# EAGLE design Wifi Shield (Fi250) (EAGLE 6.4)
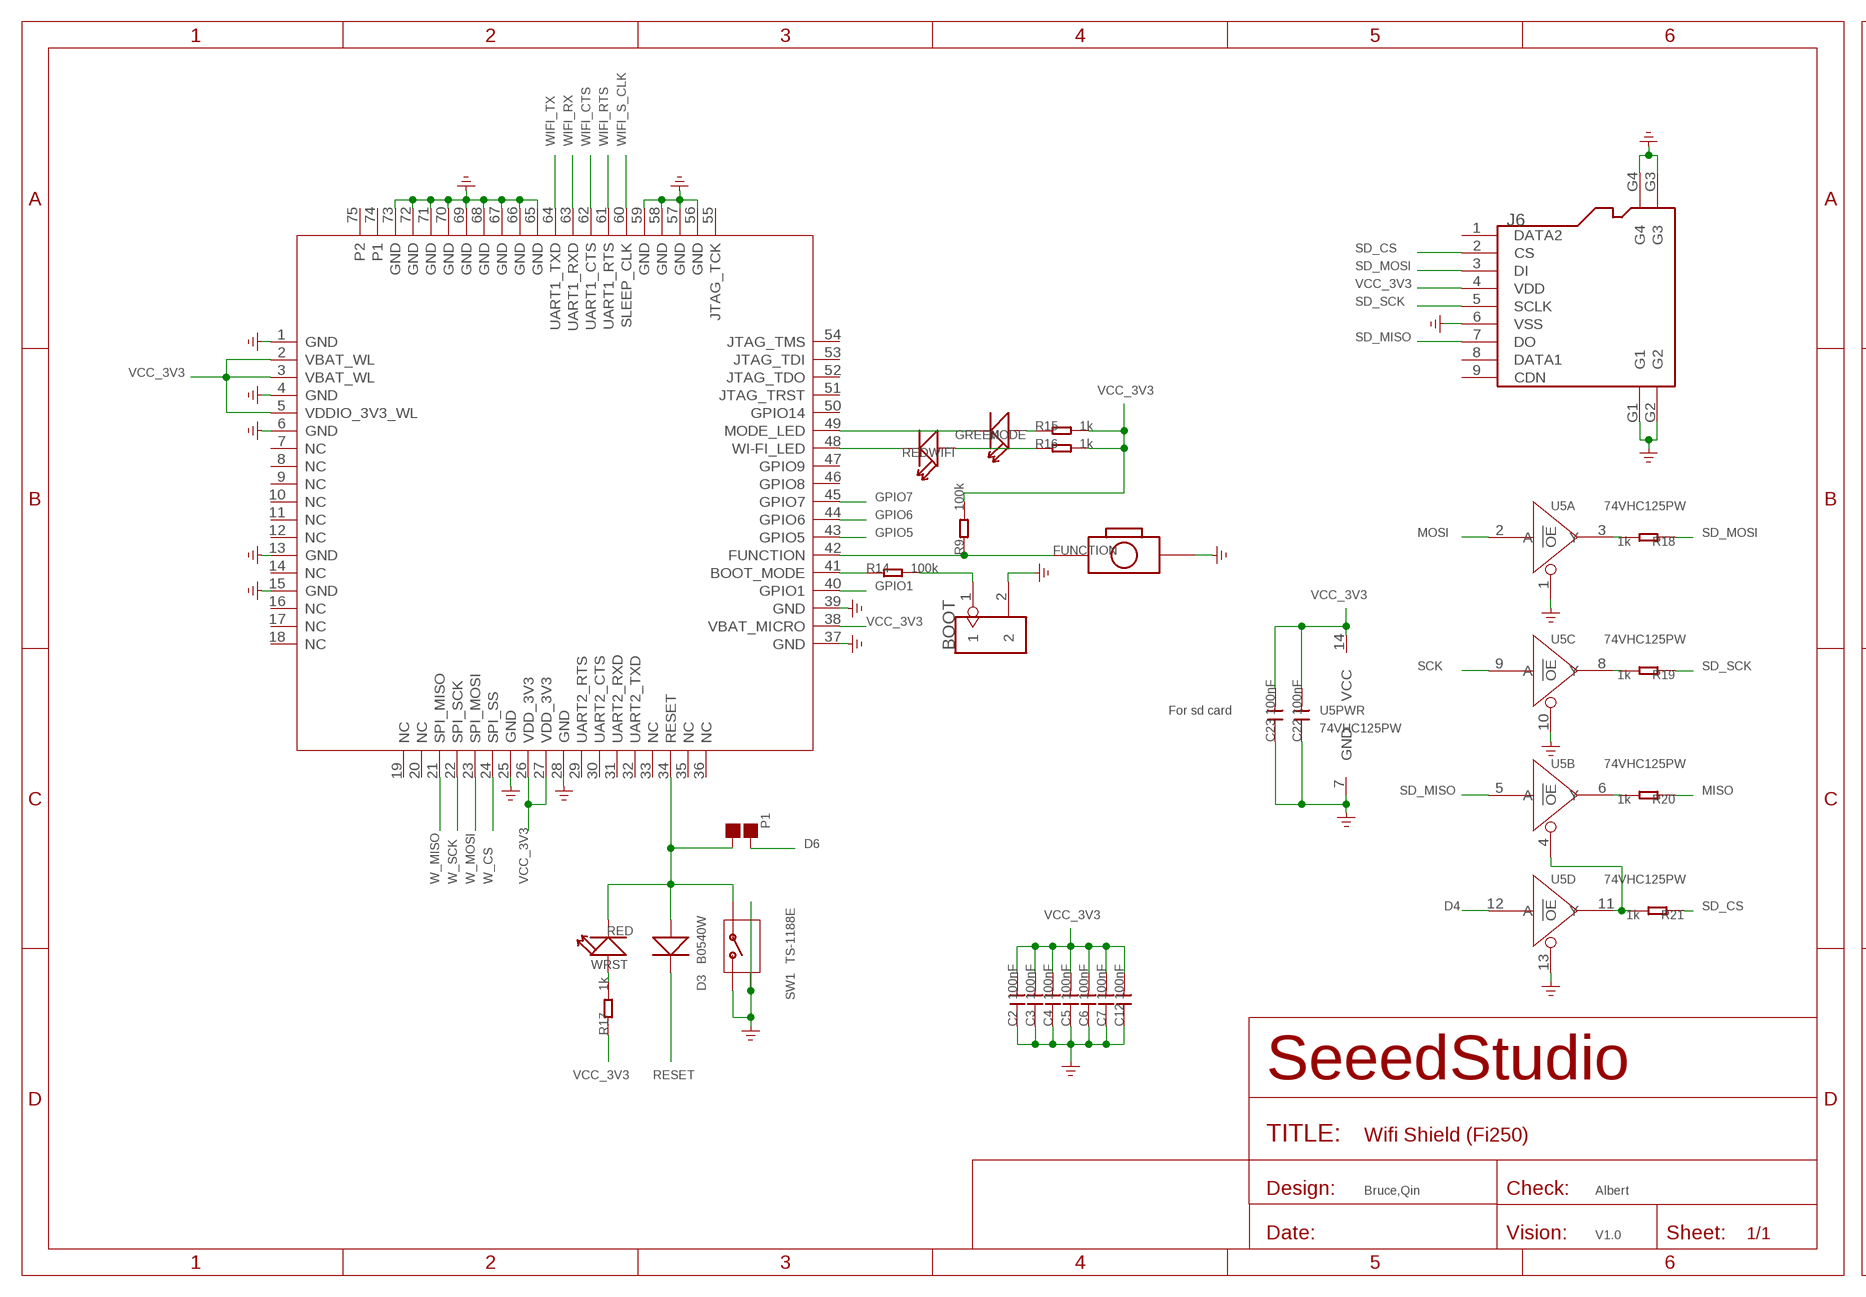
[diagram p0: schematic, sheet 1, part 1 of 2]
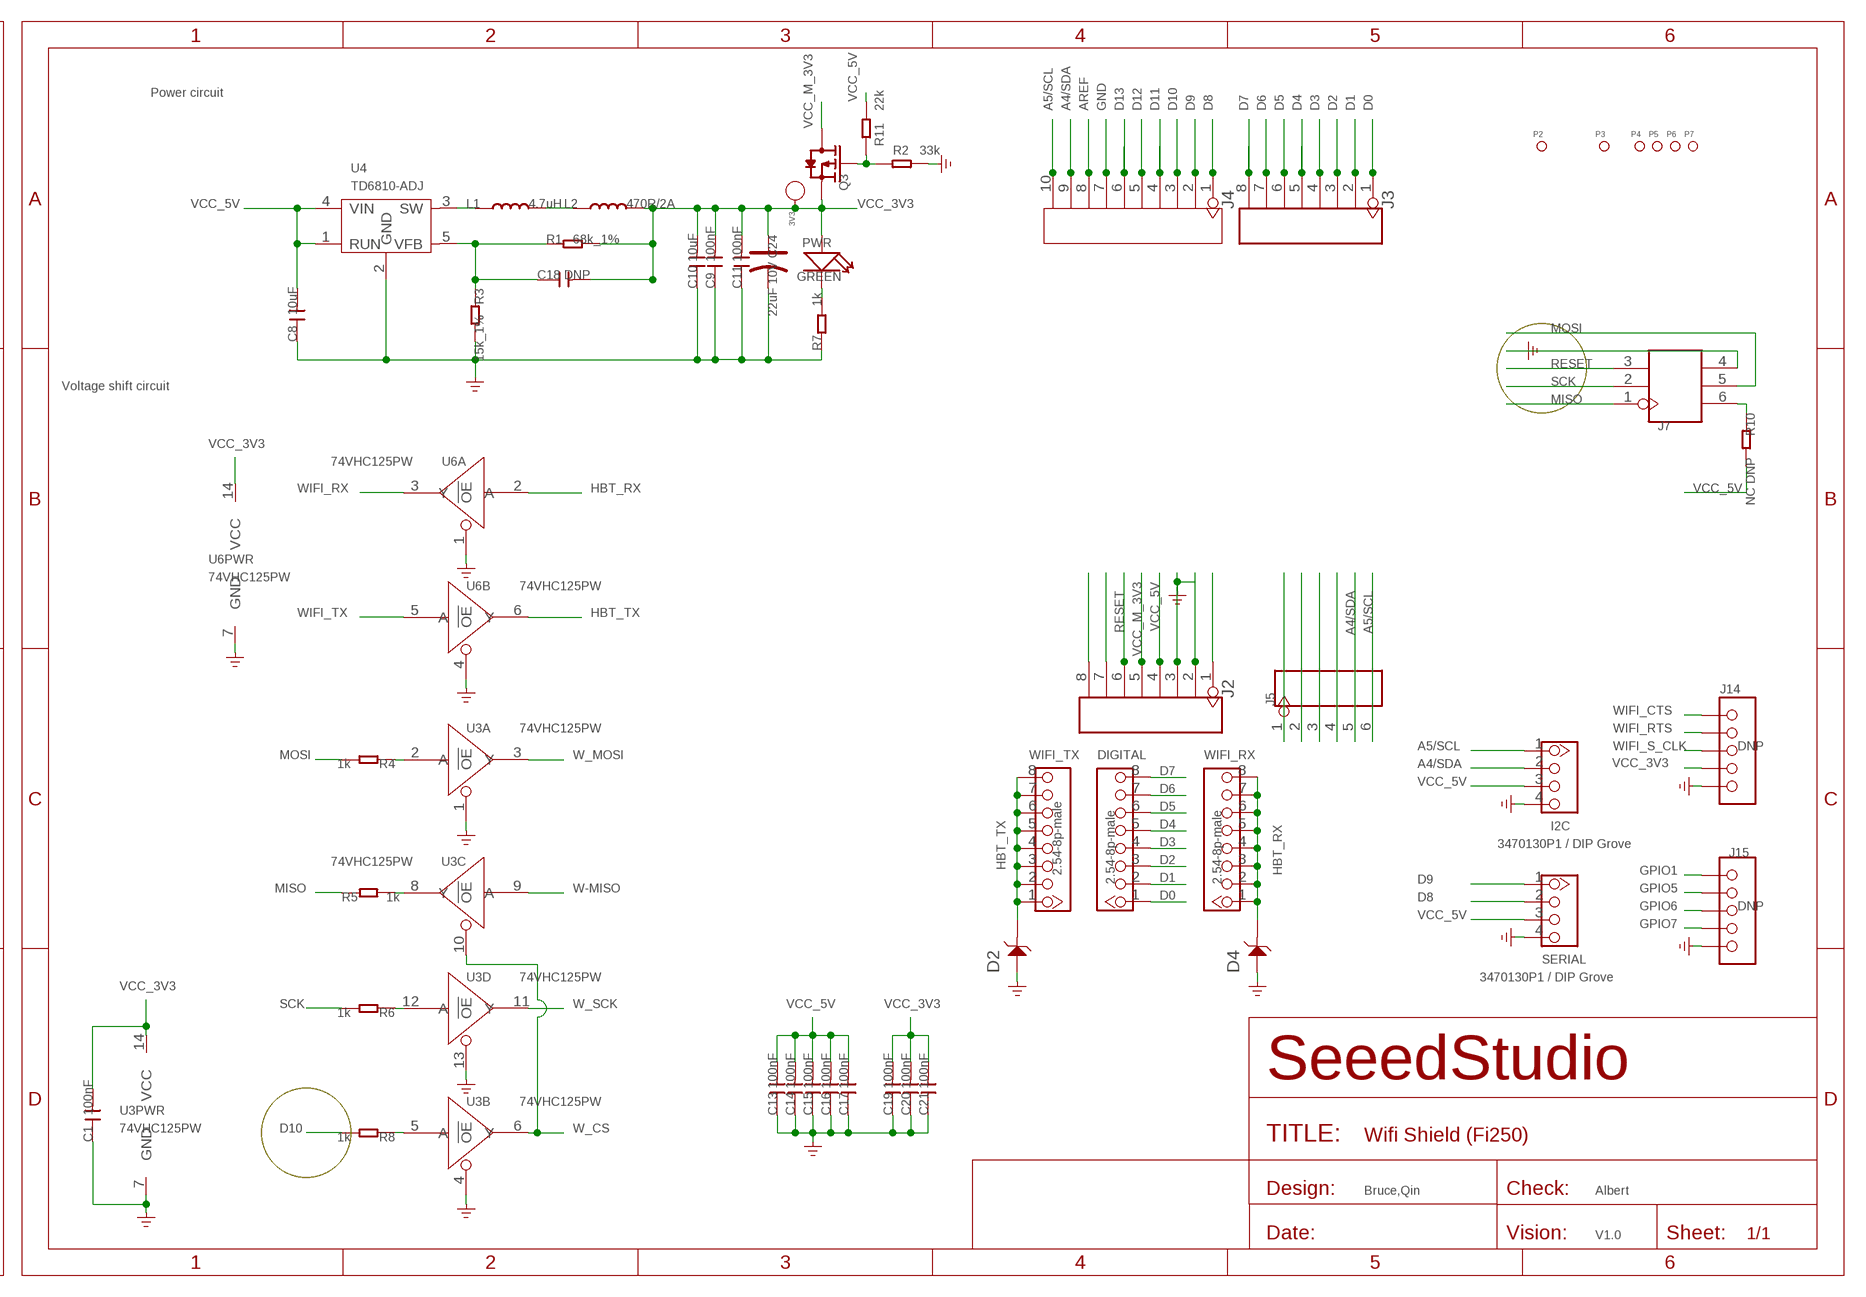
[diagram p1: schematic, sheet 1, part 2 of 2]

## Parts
3V3  PAD-TEST-POINT'4545'  [TP_4545]
BOOT  HEADER-2P-65/35MIL  [2P-2.54-65/35MIL]
C1  100nF  C-0603  [C0603]
C2  100nF  C-0603  [C0603]
C3  100nF  C-0603  [C0603]
C4  100nF  C-0603  [C0603]
C5  100nF  C-0603  [C0603]
C6  100nF  C-0603  [C0603]
C7  100nF  C-0603  [C0603]
C8  10uF  C-0805  [C0805]
C9  100nF  C-0603  [C0603]
C10  10uF  C-0805  [C0805]
C11  100nF  C-0603  [C0603]
C12  100nF  C-0603  [C0603]
C13  100nF  C-0603  [C0603]
C14  100nF  C-0603  [C0603]
C15  100nF  C-0603  [C0603]
C16  100nF  C-0603  [C0603]
C17  100nF  C-0603  [C0603]
C18  DNP  C-0603  [C0603]
C19  100nF  C-0603  [C0603]
C20  100nF  C-0603  [C0603]
C21  100nF  C-0603  [C0603]
C22  100nF  C-0603  [C0603]
C23  100nF  C-0603  [C0603]
C24  22uF 10V  CAP-AVX-A  [AVX-A]
D2  D-ESD-2P'CESD5V0D1'  [SOD123-2.7X1.6]
D3  B0540W  D'1206'  [SOD123]
D4  D-ESD-2P'CESD5V0D1'  [SOD123-2.7X1.6]
DIGITAL  2.54-8p-male  HEADER-8P-2.54  [8P-2.54]
FUNCTION  BUTTON-2P-SMD  [2P-SMD-6.1X3.81]
I2C  3470130P1 / DIP Grove  TWIG-4P-2.0-2.0  [4P-2.0]
J2  HEADER-8P-65/35MIL  [8P-2.54-65/35MIL]
J3  HEADER-8P-65/35MIL  [8P-2.54-65/35MIL]
J4  HEADER-10P-2.54  [10P-2.54]
J5  HEADER-6P-65/35MIL  [6P-2.54-65/35MIL]
J6  HOLDER-MICROSD-9P  [9P-SMD-W/-RING]
J7  HEADER-2X3P-65/35MIL  [2X3P-2.54-65/35MIL]
J14  DNP  HEADER-5P-2.54  [5P-2.54]
J15  DNP  HEADER-5P-2.54  [5P-2.54]
L1  4.7uH  LSPD3D16-4R7M  [L0420]
L2  470R/2A  L'0805'  [L0805]
MODE  GREEN  LED'0603'  [LED-0603]
P1  DNP  PAD-JUMPER-2P  [2P-SMD-1.78X1.27]
P2  PAD-MARK  [ROUND-MARK-1.0]
P3  PAD-MARK  [ROUND-MARK-1.0]
P4  PAD-MARK  [ROUND-MARK-1.0]
P5  PAD-MARK  [ROUND-MARK-1.0]
P6  PAD-MARK  [ROUND-MARK-1.0]
P7  PAD-MARK  [ROUND-MARK-1.0]
PWR  GREEN  LED'0603'  [LED-0603]
Q3  MOSFET-P'SI2323CDS/SI2305DS<BR>'  [SOT23]
R1  68k_1%  R-0603  [R0603]
R2  33k  R-0603  [R0603]
R3  15k_1%  R-0603  [R0603]
R4  1k  R-0603  [R0603]
R5  1k  R-0603  [R0603]
R6  1k  R-0603  [R0603]
R7  1k  R-0603  [R0603]
R8  1k  R-0603  [R0603]
R9  100k  R-0603  [R0603]
R10  NC DNP  R-0603  [R0603]
R11  22k  R-0603  [R0603]
R14  100k  R-0603  [R0603]
R15  1k  R-0603  [R0603]
R16  1k  R-0603  [R0603]
R17  1k  R-0603  [R0603]
R18  1k  R-0603  [R0603]
R19  1k  R-0603  [R0603]
R20  1k  R-0603  [R0603]
R21  1k  R-0603  [R0603]
SERIAL  3470130P1 / DIP Grove  TWIG-4P-2.0-2.0  [4P-2.0]
SW1  TS-1188E  BUTTON-4P-REINFORCE'TS-1188E'  [4P-SMD-7X3.5X3.5H]
U1  WIZFI250  [73P-28X20MM]
U3  74VHC125PW  74VHCT125PW  [TSSOP14]
U4  TD6810-ADJ  TD6810'TSOT23-5'  [SOT23-5]
U5  74VHC125PW  [TSSOP14]
U6  74VHC125PW  [TSSOP14]
WIFI  RED  LED'0603'  [LED-0603]
WIFI_RX  2.54-8p-male  HEADER-8P-2.54  [8P-2.54]
WIFI_TX  2.54-8p-male  HEADER-8P-2.54  [8P-2.54]
WRST  RED  LED'0603'  [LED-0603]

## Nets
A4/SDA: I2C.2 J4.9 J5.5
A5/SCL: I2C.1 J4.10 J5.6
AREF: J4.8
D0: DIGITAL.1 J3.1
D1: DIGITAL.2 J3.2
D2: DIGITAL.3 J3.3
D3: DIGITAL.4 J3.4
D4: DIGITAL.5 J3.5 U5.12(D:A)
D5: DIGITAL.6 J3.6
D6: DIGITAL.7 J3.7 P1.2
D7: DIGITAL.8 J3.8
D8: J4.1 SERIAL.2
D9: J4.2 SERIAL.1
D10: J4.3 R8.2
D11: J4.4
D12: J4.5
D13: J4.6
GND: BOOT.2 C1.1 C2.1 C3.1 C4.1 C5.1 C6.1 C7.1 C8.1 C9.1 C10.1 C11.1 C12.1 C13.1 C14.1 C15.1 C16.1 C17.1 C19.1 C20.1 C21.1 C22.1 C23.1 C24.- D2.1 D4.1 FUNCTION.P$2 I2C.4 J2.2 J2.3 J4.7 J6.6(VSS) J6.G1 J6.G2 J6.G3 J6.G4 J7.4 J14.5 J15.5 R2.1 R3.2 R7.1 SERIAL.4 SW1.2 SW1.S1 SW1.S2 U1.1(GND) U1.4(GND) U1.6(GND) U1.13(GND) U1.15(GND) U1.25(GND) U1.28(GND) U1.37(GND) U1.39(GND) U1.56(GND) U1.57(GND) U1.58(GND) U1.59(GND) U1.65(GND) U1.66(GND) U1.67(GND) U1.68(GND) U1.69(GND) U1.70(GND) U1.71(GND) U1.72(GND) U1.73(GND) U3.1(A:!OE) U3.4(B:!OE) U3.7(PWR:GND) U3.13(D:!OE) U4.2(GND) U5.1(A:!OE) U5.7(PWR:GND) U5.10(C:!OE) U5.13(D:!OE) U6.1(A:!OE) U6.4(B:!OE) U6.7(PWR:GND)
GPIO1: J15.1 U1.40(GPIO1)
GPIO5: J15.2 U1.43(GPIO5)
GPIO6: J15.3 U1.44(GPIO6)
GPIO7: J15.4 U1.45(GPIO7)
HBT_RX: D4.2 U6.2(A:A) WIFI_RX.1 WIFI_RX.2 WIFI_RX.3 WIFI_RX.4 WIFI_RX.5 WIFI_RX.6 WIFI_RX.7 WIFI_RX.8
HBT_TX: D2.2 U6.6(B:Y) WIFI_TX.1 WIFI_TX.2 WIFI_TX.3 WIFI_TX.4 WIFI_TX.5 WIFI_TX.6 WIFI_TX.7 WIFI_TX.8
MISO: J7.1 R5.1 R20.1
MOSI: J7.5 R4.2 U5.2(A:A)
N$1: J2.1
N$2: J2.7
N$3: R4.1 U3.2(A:A)
N$4: R6.1 U3.12(D:A)
N$5: J7.6 R10.1
N$6: R5.2 U3.8(C:Y)
N$7: FUNCTION.1 R9.1 U1.42(FUNCTION)
N$8: L1.1 U4.3(SW)
N$9: R17.2 WRST.+
N$10: L1.2 L2.1
N$11: J2.8
N$12: MODE.- U1.49(MODE_LED)
N$13: U1.48(WI-FI_LED) WIFI.-
N$14: BOOT.1 R14.2
N$15: R16.1 WIFI.+
N$16: J5.1
N$17: J5.2
N$18: MODE.+ R15.1
N$19: R14.1 U1.41(BOOT_MODE)
N$20: D3.+ P1.1 SW1.1 U1.34(RESET) WRST.-
N$21: J5.3
N$22: J5.4
N$23: Q3.1(G) R2.2 R11.2
N$24: R18.2 U5.3(A:Y)
N$26: PWR.- R7.2
N$27: R8.1 U3.5(B:A)
N$28: R19.2 U5.8(C:Y)
N$29: R20.2 U5.6(B:Y)
N$30: R21.2 U5.4(B:!OE) U5.11(D:Y)
N$39: C18.1 R1.1 R3.1 U4.5(VFB)
RESET: D3.- J2.6 J7.3
SCK: J7.2 R6.2 U5.9(C:A)
SD_CS: J6.2(CS) R21.1
SD_MISO: J6.7(DO) U5.5(B:A)
SD_MOSI: J6.3(DI) R18.1
SD_SCK: J6.5(SCLK) R19.1
VCC_3V3: 3V3.T C1.2 C2.2 C3.2 C4.2 C5.2 C6.2 C7.2 C9.2 C10.2 C11.2 C12.2 C18.2 C19.2 C20.2 C21.2 C22.2 C23.2 C24.+ J6.4(VDD) J14.4 L2.2 PWR.+ Q3.2(S) R1.2 R9.2 R15.2 R16.2 R17.1 U1.2(VBAT_WL) U1.3(VBAT_WL) U1.5(VDDIO_3V3_WL) U1.26(VDD_3V3) U1.27(VDD_3V3) U1.38(VBAT_MICRO) U3.14(PWR:VCC) U5.14(PWR:VCC) U6.14(PWR:VCC)
VCC_5V: C8.2 C13.2 C14.2 C15.2 C16.2 C17.2 I2C.3 J2.4 R10.2 R11.1 SERIAL.3 U4.1(RUN) U4.4(VIN)
VCC_M_3V3: J2.5 Q3.3(D)
W-MISO: U3.9(C:A)
W_CS: U1.24(SPI_SS) U3.6(B:Y) U3.10(C:!OE)
W_MISO: U1.21(SPI_MISO)
W_MOSI: U1.23(SPI_MOSI) U3.3(A:Y)
W_SCK: U1.22(SPI_SCK) U3.11(D:Y)
WIFI_CTS: J14.1 U1.62(UART1_CTS)
WIFI_RTS: J14.2 U1.61(UART1_RTS)
WIFI_RX: U1.63(UART1_RXD) U6.3(A:Y)
WIFI_S_CLK: J14.3 U1.60(SLEEP_CLK)
WIFI_TX: U1.64(UART1_TXD) U6.5(B:A)
Unconnected: J6.1(DATA2) J6.8(DATA1) J6.9(CDN) U1.7(NC) U1.8(NC) U1.9(NC) U1.10(NC) U1.11(NC) U1.12(NC) U1.14(NC) U1.16(NC) U1.17(NC) U1.18(NC) U1.19(NC) U1.20(NC) U1.29(UART2_RTS) U1.30(UART2_CTS) U1.31(UART2_RXD) U1.32(UART2_TXD) U1.33(NC) U1.35(NC) U1.36(NC) U1.46(GPIO8) U1.47(GPIO9) U1.50(GPIO14) U1.51(JTAG_TRST) U1.52(JTAG_TDO) U1.53(JTAG_TDI) U1.54(JTAG_TMS) U1.55(JTAG_TCK) U1.74(P1) U1.75(P2) U6.8(C:Y) U6.9(C:A) U6.10(C:!OE) U6.11(D:Y) U6.12(D:A) U6.13(D:!OE)

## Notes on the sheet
- Power circuit
- Voltage shift circuit
- For sd card
- Bruce,Qin | Albert | Bruce,Qin | Albert
- V1.0 | V1.0

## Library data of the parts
3V3 = Discrete:PAD-TEST-POINT; PARTNO: DNP
BOOT = Connector :HEADER-2P
C1-C23 = Discrete:C*: Ceramic Capacitors
C24 = Discrete:CAP*: Electrolytic Capacitors,Tantalum Capacitors and Super Capacitors
D2 D4 = Discrete:D-ESD-2P: Diodes for Protectiong against ESD
D3 = Discrete:D*
DIGITAL WIFI_RX WIFI_TX = Connector:HEADER-8P
FUNCTION = Discrete:BUTTON-2P
I2C SERIAL = Connector:TWIG-4P-2.0
J2 J3 = Connector :HEADER-8P
J4 = Connector :HEADER-10P
J5 = Connector :HEADER-6P
J6 = Connector :HOLDER-MICROSD-9P
J7 = Connector :HEADER-2X3P
J14 J15 = Connector:HEADER-5P
L1 = template:L
L2 = Discrete:L*
MODE PWR WIFI WRST = Discrete:LED*
P1 = Discrete:PAD-JUMPER-2P; PARTNO: DNP
P2-P7 = Discrete:PAD-MARK; PARTNO: DNP
Q3 = Discrete:MOSFET-P
R1-R11 R14-R21 = Discrete:R*
SW1 = Discrete:BUTTON-4P-REINFORCE: TS-1188E http://www.best-dz.com/?thread-374-2.html
U1 = template:WIZFI250: The WizFi250 provides for the highest-level integration, featuring 802.11b/g and 802.11n. It includes a 2.4 GHz WLAN CMOS power amplifier (PA) that meets the output power requirements of most handheld systems.
U3 U5 U6 = IC:74V*125: Quad Buffer/Line Driver;3-state
U4 = template:TD6810: 1.5MHz 800mA Synchronous Step-Down Regulator Dropout http://www.techcodeok.com/download/TD6810.pdf

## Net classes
0 default: width 0.152 mm, drill 0.305 mm, clearance 0.152 mm

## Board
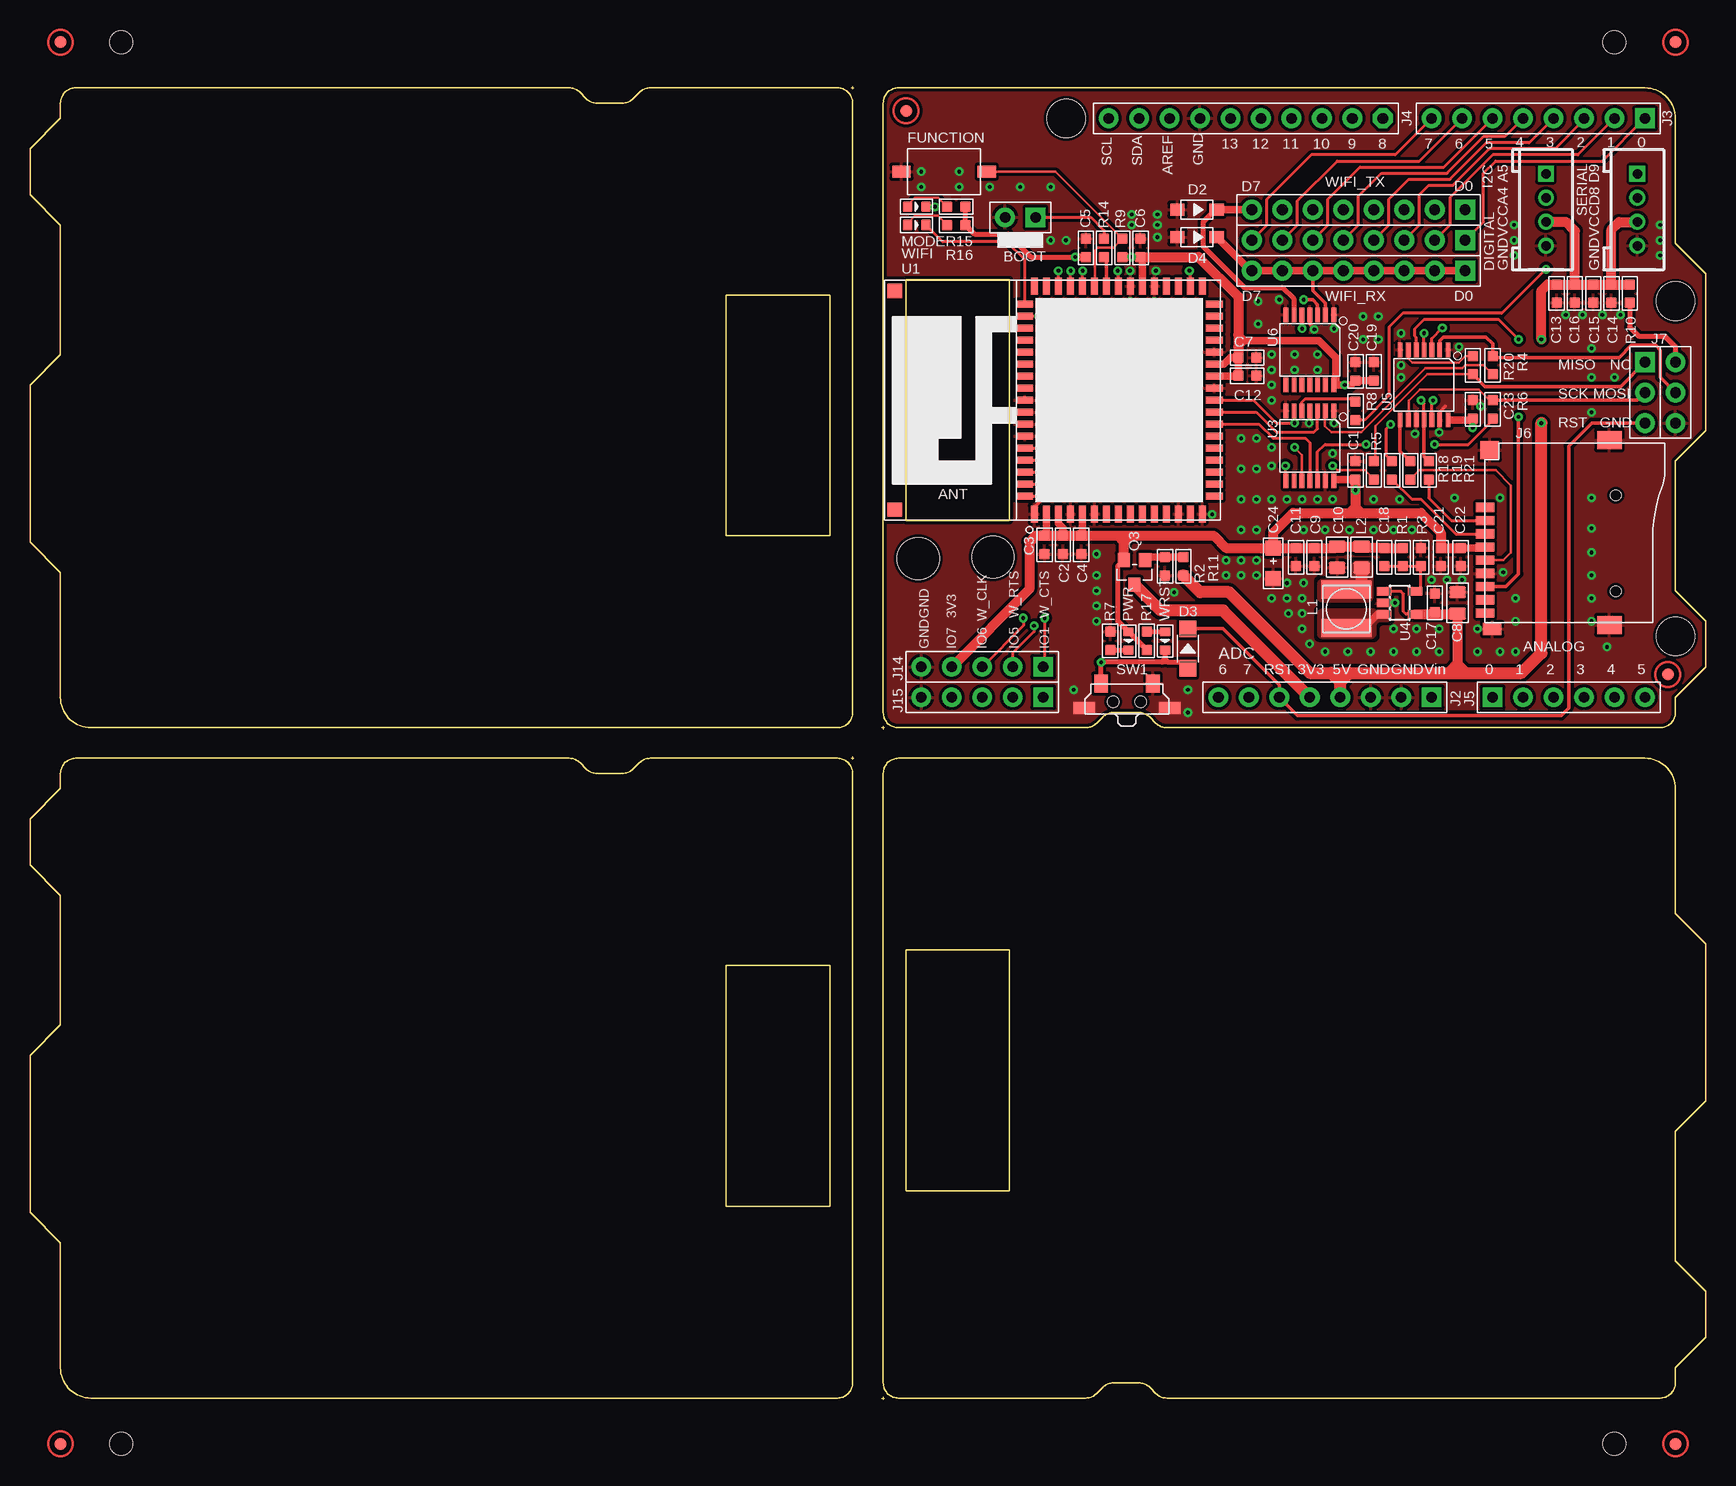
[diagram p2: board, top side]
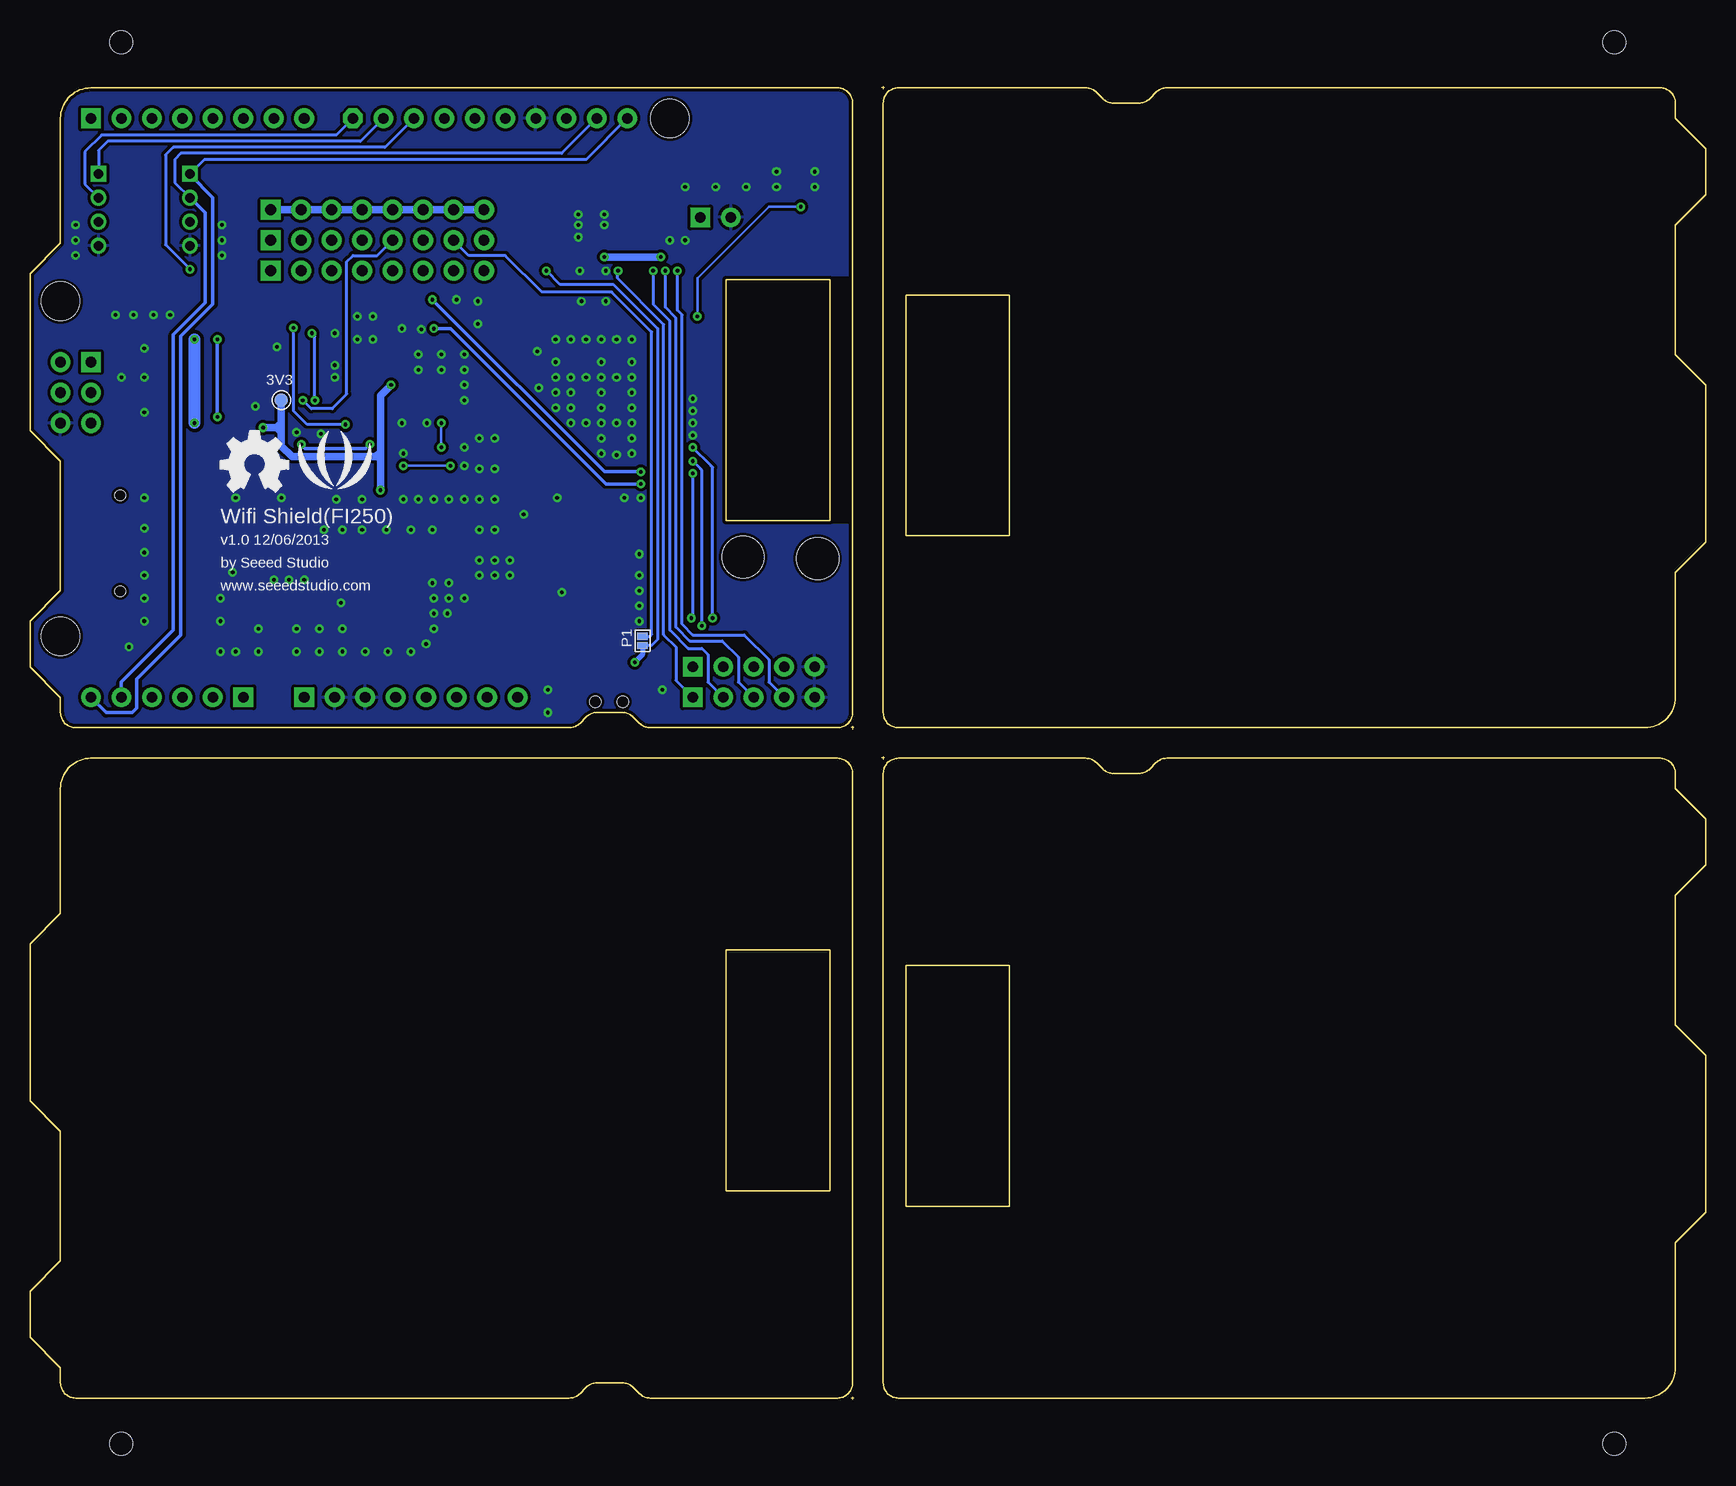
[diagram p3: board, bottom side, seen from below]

Size 139.7 x 109.47 mm. Coordinates in mm from the lower left corner, seen from the top.
Outline: 120 segments
Copper layers (1*16): Top 0.035mm / dielectric 1.5mm / Bottom 0.035mm
Design rules "default *": minimum track width 6mil, minimum drill 12mil, track to track 8mil, track to pad 8mil, pad to pad 8mil, via to via 8mil, smd to smd 0mil, copper to edge 10mil, drill to drill 8mil, minimum pad ring 10mil, minimum via ring 8mil, stop-mask expansion 4mil, vias tented up to drill 100mil, thermal gap 10mil
Holes 3.5 mm at 80.26,70.23 74.04,70.1
Holes 3.2 mm at 86.36,106.81 137.16,63.63 137.16,91.57
Holes 1.91 mm at 7.62,113.16 132.08,113.16 132.08,-3.68 7.62,-3.68
tRestrict: area 82.7,82.8 to 83.3,82.9; area 82.7,81.8 to 83.3,81.9; area 82.7,80.8 to 83.3,80.9

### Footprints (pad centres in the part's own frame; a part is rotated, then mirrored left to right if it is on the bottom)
TP_4545 = smd 1.143 x 1.143: T 0,0
2P-2.54-65/35MIL = drill 0.889 pad 1.651 square: 1 0,1.27 | drill 0.889 pad 1.651: 2 0,-1.27
C0603 = smd 0.889 x 0.889: 1 -0.762,0; 2 0.762,0
C0805 = smd 1.016 x 1.397: 1 -0.889,0; 2 0.889,0
AVX-A = smd 1.27 x 1.27: + -1.27,0; - 1.27,0
SOD123-2.7X1.6 = smd 1.2 x 1.02: 1 -1.635,0; 2 1.635,0
SOD123 = smd 1.397 x 1.397: + -1.651,0; - 1.651,0
8P-2.54 = drill 0.889 pad 1.651 square: 1 0,8.89 | drill 0.889 pad 1.651: 2 0,6.35; 3 0,3.81; 4 0,1.27; 5 0,-1.27; 6 0,-3.81; 7 0,-6.35; 8 0,-8.89
2P-SMD-6.1X3.81 = smd 1.524 x 1.016: 1 -3.556,0; P$2 3.556,0
4P-2.0 = drill 0.8 pad 1.27 square: 1 -3,0 | drill 0.8 pad 1.27: 2 -1,0; 3 1,0; 4 3,0
8P-2.54-65/35MIL = drill 0.889 pad 1.651 square: 1 0,8.89 | drill 0.889 pad 1.651: 2 0,6.35; 3 0,3.81; 4 0,1.27; 5 0,-1.27; 6 0,-3.81; 7 0,-6.35; 8 0,-8.89
10P-2.54 = drill 0.889 pad 1.651 octagon: 1 0,11.43 | drill 0.889 pad 1.651: 2 0,8.89; 3 0,6.35; 4 0,3.81; 5 0,1.27; 6 0,-1.27; 7 0,-3.81; 8 0,-6.35; 9 0,-8.89; 10 0,-11.43
6P-2.54-65/35MIL = drill 0.889 pad 1.651 square: 1 0,6.35 | drill 0.889 pad 1.651: 2 0,3.81; 3 0,1.27; 4 0,-1.27; 5 0,-3.81; 6 0,-6.35
9P-SMD-W/-RING = smd 1.524 x 0.762: 1 0,4.4; 2 0,3.3; 3 0,2.2; 4 0,1.1; 5 0,0; 6 0,-1.1; 7 0,-2.2; 8 0,-3.3; 9 0,-4.4 | smd 1.524 x 1.016: G1 0.6,-5.746 | smd 2.032 x 1.524: G2 10.373,-5.4; G3 10.373,10 | smd 1.524 x 1.524: G4 0.392,9.181 | hole 0.889: 10.9,-2.6; 10.9,5.4
2X3P-2.54-65/35MIL = drill 0.889 pad 1.651 square: 1 -1.27,2.54 | drill 0.889 pad 1.651: 2 -1.27,0; 3 -1.27,-2.54; 4 1.27,-2.54; 5 1.27,0; 6 1.27,2.54
5P-2.54 = drill 0.889 pad 1.651 square: 1 0,5.08 | drill 0.889 pad 1.651: 2 0,2.54; 3 0,0; 4 0,-2.54; 5 0,-5.08
L0420 = smd 1.5 x 4.2: 1 -1.6,0; 2 1.6,0
L0805 = smd 1.016 x 1.397: 1 -0.889,0; 2 0.889,0
LED-0603 = smd 0.762 x 0.889: + -0.762,0; - 0.762,0
2P-SMD-1.78X1.27 = smd 0.889 x 0.61: 1 0,0.381; 2 0,-0.381
ROUND-MARK-1.0 = smd 1.016 x 1.016: P$1 0,0
SOT23 = smd 1.016 x 1.143: 1 -0.889,-1.016; 2 0.889,-1.016; 3 0,1.016
R0603 = smd 0.889 x 0.889: 1 -0.762,0; 2 0.762,0
4P-SMD-7X3.5X3.5H = smd 1.143 x 1.524: 1 -2.159,1.524; 2 2.159,1.524 | smd 1.778 x 1.016: S1 -3.556,-0.508; S2 3.556,-0.508 | hole 0.95: -1.15,0; 1.15,0
73P-28X20MM = smd 0.6 x 1.4: 1 -1.5,-9.5; 2 -0.5,-9.5; 3 0.5,-9.5; 4 1.5,-9.5; 5 2.5,-9.5; 6 3.5,-9.5; 7 4.5,-9.5; 8 5.5,-9.5; 9 6.5,-9.5; 10 7.5,-9.5; 11 8.5,-9.5; 12 9.5,-9.5; 13 10.5,-9.5; 14 11.5,-9.5; 15 12.5,-9.5; 33 12.5,9.5; 34 11.5,9.5; 35 10.5,9.5; 36 9.5,9.5; 37 8.5,9.5; 38 7.5,9.5; 39 6.5,9.5; 40 5.5,9.5; 41 4.5,9.5; 42 3.5,9.5; 43 2.5,9.5; 44 1.5,9.5; 45 0.5,9.5; 46 -0.5,9.5; 47 -1.5,9.5 | smd 1.4 x 0.6: 16 13.5,-8; 17 13.5,-7; 18 13.5,-6; 19 13.5,-5; 20 13.5,-4; 21 13.5,-3; 22 13.5,-2; 23 13.5,-1; 24 13.5,0; 25 13.5,1; 26 13.5,2; 27 13.5,3; 28 13.5,4; 29 13.5,5; 30 13.5,6; 31 13.5,7; 32 13.5,8; 48 -2.3,8; 49 -2.3,7; 50 -2.3,6; 51 -2.3,5; 52 -2.3,4; 53 -2.3,3; 54 -2.3,2; 55 -2.3,1; 56 -2.3,0; 57 -2.3,-1; 58 -2.3,-2; 59 -2.3,-3; 60 -2.3,-4; 61 -2.3,-5; 62 -2.3,-6; 63 -2.3,-7; 64 -2.3,-8 | smd 1.2 x 1.2: 65 2.5,-3.5; 66 5.5,-3.5; 67 8.5,-3.5; 68 2.5,0; 69 5.5,0; 70 8.5,0; 71 2.5,3.5; 72 5.5,3.5; 73 8.5,3.5; 74 -13.12,9.12; 75 -13.12,-9.12
TSSOP14 = smd 0.4 x 1.2: 1 -2,-2.925; 2 -1.3,-2.925; 3 -0.65,-2.925; 4 0,-2.925; 5 0.65,-2.925; 6 1.3,-2.925; 7 2,-2.925; 8 2,2.925; 9 1.3,2.925; 10 0.65,2.925; 11 0,2.925; 12 -0.65,2.925; 13 -1.3,2.925; 14 -2,2.925
SOT23-5 = smd 0.69 x 1.2: 1 -0.95,-1.3; 2 0,-1.3; 3 0.95,-1.3; 4 0.95,1.3; 5 -0.95,1.3

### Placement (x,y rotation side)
3V3  118.75,83.31 0 bottom
BOOT  82.55,98.55 270 top
C1  110.49,77.47 270 top
C2  86.11,71.25 90 top
C3  84.58,71.25 90 top
C4  87.63,71.25 90 top
C5  88.01,96.01 270 top
C6  92.58,96.01 270 top
C7  101.47,86.87 180 top
C8  119,66.42 270 top
C9  107.06,70.23 90 top
C10  108.97,70.23 90 top
C11  105.54,70.23 90 top
C12  101.47,85.34 180 top
C13  127.25,92.2 90 top
C14  131.83,92.2 90 top
C15  130.3,92.2 90 top
C16  128.78,92.2 90 top
C17  117.09,66.42 270 top
C18  112.9,70.23 90 top
C19  112.01,85.72 270 top
C20  110.49,85.72 270 top
C21  117.6,70.23 90 top
C22  119.25,70.23 90 top
C23  120.27,82.55 270 top
C24  103.63,69.72 270 top
D2  97.28,99.19 0 top
D3  96.52,62.61 90 top
D4  97.28,96.9 0 top
DIGITAL  110.74,96.65 270 top
FUNCTION  76.2,102.36 180 top
I2C  126.37,99.19 270 top
J2  107.95,58.55 270 top
J3  125.73,106.81 270 top
J4  101.35,106.81 270 top
J5  128.27,58.55 90 top
J6  121.28,69.98 0 top
J7  135.89,83.95 0 top
J14  79.38,61.09 270 top
J15  79.38,58.55 270 top
L1  109.73,65.91 90 top
L2  111,70.23 90 top
MODE  73.91,99.44 0 top
P1  88.65,63.25 180 bottom
P2  73.03,107.44 0 top
P3  136.53,60.45 0 top
P4  not placed on the board
P5  not placed on the board
P6  not placed on the board
P7  not placed on the board
PWR  91.57,63.25 270 top
Q3  92.08,68.96 180 top
R1  114.43,70.23 90 top
R2  94.62,69.47 90 top
R3  115.95,70.23 90 top
R4  121.92,86.23 90 top
R5  112.01,77.47 270 top
R6  121.92,82.55 90 top
R7  90.04,63.25 270 top
R8  110.49,82.42 270 top
R9  91.06,96.01 270 top
R10  133.35,92.2 90 top
R11  96.14,69.47 90 top
R14  89.53,96.01 90 top
R15  77.22,99.44 0 top
R16  77.22,97.92 0 top
R17  93.09,63.25 90 top
R18  113.54,77.47 90 top
R19  115.06,77.47 90 top
R20  120.27,86.23 90 top
R21  116.59,77.47 90 top
SERIAL  133.99,99.19 270 top
SW1  91.44,58.17 0 top
U1  85.22,83.31 0 top
U3  106.68,79.5 180 top
U4  114.17,66.42 270 top
U5  116.21,84.58 180 top
U6  106.68,87.5 180 top
U$23  [OSHW_FILLX200_NOTEXT]  123.83,75.69 0 bottom
U$24  [LOGO_SILK]  114.3,77.6 0 bottom
WIFI  73.91,97.92 0 top
WIFI_RX  110.74,94.11 270 top
WIFI_TX  110.74,99.19 270 top
WRST  94.62,63.25 270 top

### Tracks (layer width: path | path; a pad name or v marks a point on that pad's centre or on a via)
A4/SDA
  Bottom 0.254: J4.9 95.38,103.89 127.13,103.89 127.64,103.38 127.64,101.46 I2C.2
  Bottom 0.305: I2C.2 126.35,100.19 125.09,98.93 125.09,91.44 127.76,88.77 127.76,64.13 132.08,59.82 J5.5
A5/SCL
  Bottom 0.254: J4.10 93.34,103.38 125.17,103.38 I2C.1
  Bottom 0.305: I2C.1 126.37,102.11 124.46,100.2 124.46,91.31 127.13,88.65 127.13,63.75 130.81,60.07 130.81,57.66 131.19,57.28 133.35,57.28 J5.6
D0
  Top 0.254: DIGITAL.1 121.16,98.17 121.16,102.23 122.18,103.25 131.06,103.25 J3.1
D1
  Top 0.254: DIGITAL.2 118.36,97.92 118.36,100.2 121.92,103.76 129.03,103.76 J3.2
D2
  Top 0.254: J3.3 129.54,106.68 127.13,104.27 121.67,104.27 118.62,101.22 116.59,101.22 115.82,100.46 115.82,97.92 DIGITAL.3
D3
  Top 0.254: J3.4 124.97,104.78 121.41,104.78 118.36,101.73 114.94,101.73 113.28,100.08 113.28,97.92 DIGITAL.4
D4  (via drill 0.3 pad 0.64)
  Top 0.254: J3.5 122.94,105.28 121.16,105.28 118.11,102.23 112.65,102.23 110.74,100.33 110.74,97.92 DIGITAL.5 | U5.12 116.86,83.2 v116.97,83.31
  Bottom 0.254: DIGITAL.5 110.74,95.38 112.78,95.38 113.28,94.87 113.28,83.82 114.51,82.59 116.25,82.59 v116.97,83.31
D5
  Top 0.254: J3.6 117.86,102.74 110.87,102.74 108.2,100.08 108.2,97.92 DIGITAL.6
D6
  Top 0.254: DIGITAL.7 105.66,97.92 105.66,99.94 108.98,103.25 115.82,103.25 J3.7
  Bottom 0.254: P1.2 88.06,63.63 87.88,63.81 87.88,89 91.22,92.33 97.03,92.33 100.08,95.38 103.12,95.38 DIGITAL.7
D7
  Top 0.254: DIGITAL.8 103.12,97.92 103.12,100.08 106.81,103.76 113.79,103.76 J3.8
D8
  Bottom 0.254: SERIAL.2 135.13,101.33 135.13,104.01 133.73,105.41 114.17,105.41 J4.1
D9
  Bottom 0.254: J4.2 112.14,104.9 133.22,104.9 133.99,104.14 SERIAL.1
D10  (via drill 0.3 pad 0.64)
  Top 0.254: v126.37,94.23 122.68,90.55 114.43,90.55 113.28,89.41 113.28,83.69 111.25,81.66 R8.2
  Bottom 0.254: J4.3 110.11,104.39 127.76,104.39 128.4,103.76 128.4,96.27 v126.37,94.23
GND  (via drill 0.3 pad 0.64)
  Top 0.254: U3.4 106.68,81.47 v106.62,81.41
  Top 0.305: U6.4 106.68,89.66 107.06,89.28 | U1.1 83.72,74.38 84.58,75.25 88.71,75.25 v88.77,75.18 | U5.13 117.5,82.33 117.98,82.8
  other vias: 86.36,96.65 85.09,96.65 91.82,97.92 91.82,98.81 93.98,98.81 93.98,97.92 93.98,96.9 128.02,90.42 129.41,90.42 131.06,90.42 132.59,90.42 120.9,82.8 103.5,87.12 103.5,85.85 105.41,87.12 105.41,85.85 107.31,87.12 107.31,85.85 103.5,84.58 103.5,83.31 103.5,77.85 103.5,79.38 108.59,78.87 112.4,88.39 111.12,88.39 111.12,90.3 112.4,90.3 104.78,66.8 106.05,66.8 106.17,68.07 104.78,68.07 106.05,65.53 104.9,65.53 106.05,64.26 106.68,62.99 107.95,62.36 109.86,62.36 111.76,62.36 113.67,62.36 115.57,62.36 117.47,62.36 117.47,64.26 115.57,64.26 113.67,64.26 113.79,66.42 116.84,68.33 118.11,68.33 119.38,68.33 103.5,66.8 102.23,68.71 102.23,69.98 100.97,69.98 99.7,69.98 99.7,68.71 100.97,68.71 109.98,72.52 112.01,72.52 107.95,72.52 106.17,72.52 113.67,72.52 115.19,72.52 95.38,67.31 88.9,70.48 88.9,68.71 88.9,67.44 88.9,66.17 88.9,64.9 96.52,59.18 96.52,57.28 87,59.18 102.23,72.52 100.97,72.52 100.97,75.06 102.23,75.06 102.23,77.6 100.97,77.6 100.97,80.14 102.23,80.14 106.05,75.06 108.59,75.06 112.01,75.06 114.17,75.06 118.75,75.18 122.56,75.18 130.18,75.18 130.18,72.64 130.18,70.61 130.18,68.71 130.18,66.8 130.18,64.9 123.83,64.9 123.83,66.8 122.81,68.96 120.65,62.36 120.65,64.26 122.56,62.36 123.83,62.36 131.44,62.74 132.08,85.22 130.18,85.22 130.18,82.3 130.18,87.63 114.3,86.23 114.3,85.22 114.3,88.9 108.71,89.28 104.14,91.69 102.36,91.57 102.36,89.66 107.31,75.06 104.78,75.06 103.5,75.06 119.13,87.76 107.06,89.22 90.81,88.39 89.53,88.39 89.53,86.49 89.53,85.22 90.81,85.22 92.08,85.22 92.08,86.49 92.08,88.39 89.53,83.95 92.08,83.95 92.08,82.68 89.53,82.68 89.53,81.41 90.81,81.41 92.08,81.41 92.08,80.14 92.08,78.87 90.81,78.74 89.53,78.87 89.53,80.14 93.34,81.41 94.62,81.41 93.34,85.22 93.34,88.39 94.62,88.39 94.62,85.22 95.89,85.22 95.89,86.49 95.89,88.39 95.89,83.95 95.89,82.68 94.62,83.95 94.62,82.68 90.17,75.18 93.85,94.11 91.69,94.11 97.41,87.38 97.28,84.33 95.76,75.18 98.55,73.79 91.69,91.57 93.73,91.57 84.46,80.39 84.46,82.42 84.46,81.41 84.46,83.44 74.3,102.36 74.3,101.09 77.47,101.09 77.47,102.36 80.01,101.09 82.55,101.09 85.09,101.09 115.44,80.52 117.47,80.64 108.71,81.41 123.7,96.65 123.7,95.38 123.7,97.92 135.89,97.92 135.89,96.65 135.89,95.38
  pour Bottom (isolate 0.254, rank 6): 71.12,109.98 139.7,109.98 139.7,56.01 71.12,56.01 71.12,72.9 73.03,72.9 73.03,93.73 71.12,93.73
  pour Top (isolate 0.254, rank 6): 71.12,109.98 139.7,109.98 139.7,56.01 71.12,56.01 71.12,72.9 73.03,72.9 73.03,93.73 71.12,93.73
GPIO1  (via drill 0.3 pad 0.64)
  Top 0.254: U1.40 90.72,94.07 v90.68,94.11
  Bottom 0.254: J15.1 85.85,59.94 85.85,62.74 86.87,63.75 86.87,89.62 90.72,93.47 90.72,94.07 v90.68,94.11
GPIO5  (via drill 0.3 pad 0.64)
  Top 0.254: U1.43 87.72,94.07 v87.76,94.11
  Bottom 0.254: J15.2 83.19,59.82 83.19,62.1 83.69,62.61 84.84,62.61 86.36,64.13 86.36,89.92 87.76,91.31 v87.76,94.11
GPIO6  (via drill 0.3 pad 0.64)
  Top 0.254: U1.44 86.72,94.08 v86.74,94.11
  Bottom 0.254: J15.3 80.65,59.82 80.65,61.89 82,63.25 84.71,63.25 85.85,64.39 85.85,90.17 86.74,91.06 v86.74,94.11
GPIO7  (via drill 0.3 pad 0.64)
  Top 0.254: U1.45 85.72,94.1 v85.73,94.11
  Bottom 0.254: J15.4 78.11,59.82 78.11,61.69 80.17,63.75 84.46,63.75 85.34,64.64 85.34,90.42 85.73,90.81 85.73,93.97 85.72,93.98 v85.72,94.1 v85.73,94.11
HBT_RX
  Top 0.305: U6.2 107.98,91.41 106.93,92.46 WIFI_RX.6
  Top 0.61: D4.2 101.71,94.11 WIFI_RX.8 WIFI_RX.7 WIFI_RX.6 WIFI_RX.5 WIFI_RX.4 WIFI_RX.3 WIFI_RX.2 WIFI_RX.1
HBT_TX
  Top 0.406: D2.2 98.81,99.19 97.79,98.17 97.79,96.14 101.22,92.71 104.39,92.71 105.38,91.72 105.38,91.66 U6.6
  Top 0.61: WIFI_TX.8 D2.2
  Bottom 0.61: WIFI_TX.8 WIFI_TX.7 WIFI_TX.6 WIFI_TX.5 WIFI_TX.4 WIFI_TX.3 WIFI_TX.2 WIFI_TX.1
MISO
  Top 0.203: R20.1 116.46,85.47 112.14,81.15 112.14,78.36 R5.1
  Top 0.305: J7.1 132.59,84.45 121.28,84.45 R20.1
MOSI
  Top 0.305: U5.2 117.5,88.29 117.8,88.58 121.35,88.58 121.92,88.01 R4.2 122.05,86.87 132.46,86.87 133.48,87.88 135.51,87.88 135.89,87.5 135.89,85.22 J7.5
N$3
  Top 0.203: R4.1 121.16,86.23 119.63,86.23 119.38,85.98 116.33,85.98 110.99,80.63 108.47,80.63 107.95,81.15 107.95,82.4 U3.2
N$4  (via drill 0.3 pad 0.64)
  Top 0.254: U3.12 107.33,79.01 107.95,79.63 v111.38,79.63 | v117.09,79.63 119.89,79.63 121.79,81.53 121.79,81.66 R6.1
  Bottom 0.305: v111.38,79.63 111.72,79.29 116.76,79.29 v117.09,79.63
N$5
  Top 0.406: R10.1 133.35,89.41 134.11,88.65 136.27,88.65 137.16,87.76 J7.6
N$6  (via drill 0.3 pad 0.64)
  Top 0.203: v104.65,77.85 104.65,76.61 U3.8 | R5.2 111.25,77.47 108.97,77.47 v108.59,77.85
  Bottom 0.203: v104.65,77.85 v108.59,77.85
N$7
  Top 0.203: U1.42 88.75,92.81 88.77,92.84 88.77,95.76 89.03,96.01 90.3,96.01 R9.1 85.47,102.36 FUNCTION.1
N$8
  Top 0.61: U4.3 112.33,65.47 111.25,64.39 109.8,64.39 L1.1
  pour Top (isolate 0.254, no thermals): 107.76,65.85 113.27,65.85 arc-90 113.41,65.71 113.41,65.28 arc-90 113.03,64.9 112.52,64.9 arc90 112.14,64.52 112.14,63.88 arc-90 111.76,63.5 107.76,63.5 arc-90 107.38,63.88 107.38,65.47 arc-90
N$9
  Top 0.406: R17.2 WRST.+
N$10
  Top 1.016: L2.1 111,67.94 110.49,67.44 109.73,67.44 109.6,67.56 109.68,67.56 L1.2
  pour Top (isolate 0.254, no thermals): 110.24,68.71 110.24,69.47 arc-90 110.62,69.85 111.51,69.85 arc-90 111.89,69.47 111.89,66.93 arc-90 111.51,66.55 107.76,66.55 arc-90 107.38,66.93 107.38,67.94 arc-90 107.76,68.33 109.86,68.33 arc90
N$12  (via drill 0.3 pad 0.64)
  Top 0.203: U1.49 84.06,90.31 v84.07,90.3 | MODE.- v75.44,99.44
  Bottom 0.203: v84.07,90.3 84.07,93.47 78.11,99.44 v75.44,99.44
N$13
  Top 0.254: U1.48 82.92,95.01 81.41,96.52 76.07,96.52 WIFI.-
N$14
  Top 0.254: R14.2 89.53,97.45 88.44,98.55 BOOT.1
N$15
  Top 0.203: WIFI.+ 73.15,98.04 73.79,98.68 75.69,98.68 R16.1
N$18
  Top 0.203: MODE.+ 73.15,99.57 73.79,100.2 75.69,100.2 R15.1
N$19
  Top 0.305: 89.59,95.19 R14.1 89.72,95.07 U1.41
N$20  (via drill 0.3 pad 0.64)
  Top 0.254: U1.34 96.72,94.04 v96.65,94.11
  Top 0.406: 94.87,61.47 94.36,61.47 | 94.36,61.47 v89.28,61.47 SW1.1 | WRST.- 94.62,61.72 | 94.62,61.72 94.36,61.47 | 94.62,61.72 94.87,61.47 | 94.87,61.47 96.01,61.47 D3.+
  Bottom 0.254: P1.1 87.88,62.86 87.38,63.37 87.38,89.28 91.06,92.96 95.5,92.96 v96.65,94.11
  Bottom 0.406: P1.1 88.65,62.1 v89.28,61.47
N$23
  Top 0.61: Q3.1 93.22,70.23 R2.2 R11.2
N$24  (via drill 0.3 pad 0.64)
  Top 0.203: 116.84,87.52 U5.3
  Top 0.254: R18.2 113.03,78.74 113.03,80.9 v113.41,81.28 | 116.84,87.52 116.84,88.46 v117.73,89.34
  Bottom 0.254: v113.41,81.28 116.59,81.28 117.73,82.42 v117.73,89.34
N$26
  Top 0.406: R7.2 PWR.-
N$27
  Top 0.254: U3.5 106.03,83.17 106.3,83.44 110.24,83.44 R8.1
N$28
  Top 0.305: U5.8 114.21,79.09 R19.2
N$29
  Top 0.203: U5.6 114.91,86.77 115.22,86.45 119.09,86.45 119.63,87 R20.2
N$30  (via drill 0.3 pad 0.64)
  Top 0.254: U5.4 v116.21,88.9 | U5.11 116.21,83.06 v115.95,83.31
  Top 0.305: U5.11 116.21,78.61 R21.2
  Bottom 0.254: v115.95,83.31 115.95,88.65 v116.21,88.9
N$39
  Top 0.254: C18.1 R1.1 R3.1 115.95,67.69 115.63,67.37 U4.5
RESET
  Top 0.305: J7.3 130.18,81.41 128.27,79.5 128.27,57.66 127.64,57.02 105.66,57.02 J2.6 104.14,59.56 99.44,64.26 D3.-
SCK
  Top 0.203: R6.2 121.67,83.31 120.78,84.2 115.85,84.2 114.94,83.28 114.94,81.69 U5.9
  Top 0.305: J7.2 133.99,83.31 R6.2
SD_CS
  Top 0.254: R21.1 116.59,75.15 118.46,73.28 J6.2
SD_MISO  (via drill 0.3 pad 0.64)
  Top 0.254: U5.5 115.56,88.53 115.44,88.65 115.44,89.29 116.22,90.06 122.41,90.06 v124.08,88.39
  Top 0.305: J6.7 123.02,67.78 124.08,68.83 v124.08,81.91
  Bottom 0.305: v124.08,81.91 v124.08,88.39
SD_MOSI
  Top 0.254: J6.3 121.24,72.14 118.87,72.14 115.95,75.06 115.19,75.06 R18.1
SD_SCK
  Top 0.203: R19.1 115.82,77.47 122.17,77.47 123.44,76.2 123.44,70.61 122.81,69.98 J6.5
VCC_3V3  (via drill 0.3 pad 0.64)
  Top 0.406: Q3.2 90.68,69.47 90.68,64.9 PWR.+ R17.1 | U5.14 118.36,81.66 | U6.14 108.84,84.58 | 108.84,76.71 108.81,76.71 U3.14 | v87.12,95.25 83.44,95.25 81.53,97.16 78.74,97.16 R16.2 R15.2
  Top 0.61: 92.46,95.25 C6.2 92.72,95.12 U1.38 | 92.46,95.25 91.95,95.25 v91.82,95.25 R9.2 | v87.12,95.25 C5.2 | U1.3 85.72,73.03 86.11,72.64 C2.2 | C19.2 C20.2 110.11,84.58 v109.6,84.58 | C22.2 121.2,70.99 J6.4 | 118.36,81.66 120.14,81.66 C23.2 v120.27,81.03 | C1.2 108.84,76.71 | 101.22,88.27 107.44,88.27 108.84,86.87 108.84,84.58 v109.6,84.58 | 101.22,88.27 100.71,88.77 | 101.22,88.27 100.71,87.76 | 92.59,95.12 92.46,95.25 | U1.2 84.72,72.02 84.71,72.01 | U1.5 87.72,72.1 C4.2 | U1.27 99.52,86.31 100.08,86.87 C7.2 C12.2 100.68,85.31 U1.26 | v109.6,84.58
  Top 0.813: C6.2 97.41,95.25 100.71,91.95 100.71,88.77 100.71,87.76 C7.2 | C24.+ C11.2 C9.2 108.84,70.99 C10.2 L2.2 111.12,70.99 C18.2 R1.2 | C22.2 C21.2 117.6,72.26 115.95,73.91 111,73.91 | C1.2 v110.49,75.82 110.49,74.42 | 110.49,74.42 110.49,73.91 | 110.49,73.91 111,73.91 | 109.98,73.91 105.28,73.91 103.63,72.26 C24.+ | 109.98,73.91 110.49,73.91 | 90.68,72.01 C4.2 C2.2 84.71,72.01 C3.2 83.82,72.01 83.31,71.5 83.31,67.56 J14.4 | 90.68,72.01 91.19,72.01 | 91.19,72.01 91.69,72.01 | 91.69,72.01 98.68,72.01 99.7,70.99 C24.+ | Q3.2 91.19,71.5 | 91.19,71.5 91.19,72.01 | 91.19,71.5 90.68,72.01 | 91.19,71.5 91.69,72.01 | 110.49,74.42 109.98,73.91 | 110.49,74.42 111,73.91
  Bottom 0.61: 110.49,78.99 110.49,78.36 | 110.49,78.36 v110.49,75.82 | 110.87,78.61 117.86,78.61 118.75,79.5 118.75,80.64 | 110.87,78.61 110.74,78.61 110.49,78.36 | 110.87,78.61 110.49,78.99 | v87.12,95.25 v91.82,95.25 | 3V3.T 118.75,81.41 | 118.75,81.41 118.75,81.03 | 118.75,81.03 118.75,80.64 | v120.27,81.03 119.13,81.03 | 119.13,81.03 118.75,81.03 | 119.13,81.03 118.75,81.41 | 119.13,81.03 118.75,80.64 | 110.49,78.99 110.49,83.69 v109.6,84.58
VCC_5V  (via drill 0.3 pad 0.64)
  Top 0.254: U4.1 114.29,67.37 114.49,67.17 114.49,65.67 114.7,65.47 U4.4
  Top 0.813: U4.4 116.91,65.47 | 116.91,65.47 C17.2 | 116.91,65.47 118.94,65.47 C8.2 119,61.34 | 119,61.34 119,60.71 119.13,60.58 | 119,61.34 118.36,60.71 | 119,61.34 119.63,60.71 | v125.98,88.39 125.98,92.46 126.49,92.96 C13.2 C16.2 | C16.2 C15.2 C14.2 | C14.2 R10.2 | C16.2 128.78,97.41 128,98.19 I2C.3 | C14.2 131.83,97.54 132.46,98.17 133.97,98.17 SERIAL.3
  Top 1.016: 108.46,60.58 106.68,60.58 99.95,67.31 97.54,67.31 R11.1 | 108.46,60.58 109.98,60.58 | 109.22,59.82 109.98,60.58 | J2.4 109.22,59.82 | 109.22,59.82 108.46,60.58 | 109.98,60.58 119.13,60.58 124.33,60.58 125.98,62.23 v125.98,81.41
  Bottom 1.016: v125.98,81.41 v125.98,88.39
VCC_M_3V3
  Top 1.016: J2.5 99.44,65.79 94.23,65.79 Q3.3
W_CS  (via drill 0.3 pad 0.64)
  Top 0.203: U3.10 106.03,78.75 v105.41,79.38
  Top 0.254: U1.24 101.98,83.31 103.89,81.41 v105.41,81.41 105.41,82.4 U3.6
  Bottom 0.203: v105.41,79.38 v105.41,81.41
W_MOSI
  Top 0.254: U1.23 102.22,82.31 103.9,80.63 107.02,80.63 107.31,80.93 107.31,82.41 U3.3
W_SCK
  Top 0.254: U1.22 102.46,81.31 103.63,80.14 106.32,80.14 106.68,79.78 U3.11
WIFI_CTS  (via drill 0.3 pad 0.64)
  Top 0.254: U1.62 84.36,77.31 v84.46,77.22 | v84.58,65.15 84.58,61.21 J14.1
  Bottom 0.254: v84.46,77.22 84.46,65.28 v84.58,65.15
WIFI_RTS  (via drill 0.3 pad 0.64)
  Top 0.254: U1.61 84.38,78.31 v84.46,78.23 | v83.69,64.52 83.69,64.01 81.92,62.23 J14.2
  Bottom 0.254: v83.69,64.52 83.69,77.47 83.82,77.6 v84.46,78.23
WIFI_RX  (via drill 0.3 pad 0.64)
  Top 0.254: 107.31,90.41 U6.3 | U1.63 87.74,76.31 v88.77,77.34
  Top 0.305: v106.17,91.69 106.93,91.69 107.33,91.3 U6.3
  Bottom 0.305: v106.17,91.69 91.82,77.34 v88.77,77.34
WIFI_S_CLK  (via drill 0.3 pad 0.64)
  Top 0.254: U1.60 84.39,79.31 v84.46,79.38 | v82.8,65.15 82.8,64.52 J14.3
  Bottom 0.254: v82.8,65.15 82.8,77.72 82.93,77.85 v84.46,79.38
WIFI_TX  (via drill 0.3 pad 0.64)
  Top 0.254: 106.05,90.41 U6.5 | U1.64 83.82,75.31 84.33,75.82 88.27,75.82 v88.77,76.33
  Top 0.305: U6.5 106.03,89.3 v106.05,89.28
  Bottom 0.305: v106.05,89.28 104.65,89.28 91.69,76.33 v88.77,76.33

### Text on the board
tPlace: 13 | 12 | 11 | 10 | 9 | 8 | 7 | 6 | 5 | 4 | 3 | 2 | 1 | 0 | SCL | SDA | GND | AREF | D7 | D0 | A5 | D9 | A4 | D8 | VCC | VCC | GND | GND | D7 | D0 | MISO | NC | SCK | MOSI | RST | GND | GND | 3V3 | W_CLK | W_RTS | W_CTS | GND | IO7 | IO6 | IO5 | IO1 | ADC | ANALOG | 6 | 7 | RST | 3V3 | 5V | GND | GND | Vin | 0 | 1 | 2 | 3 | 4 | 5
bPlace: Wifi Shield(FI250) | v1.0 12/06/2013 | by Seeed Studio | www.seeedstudio.com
